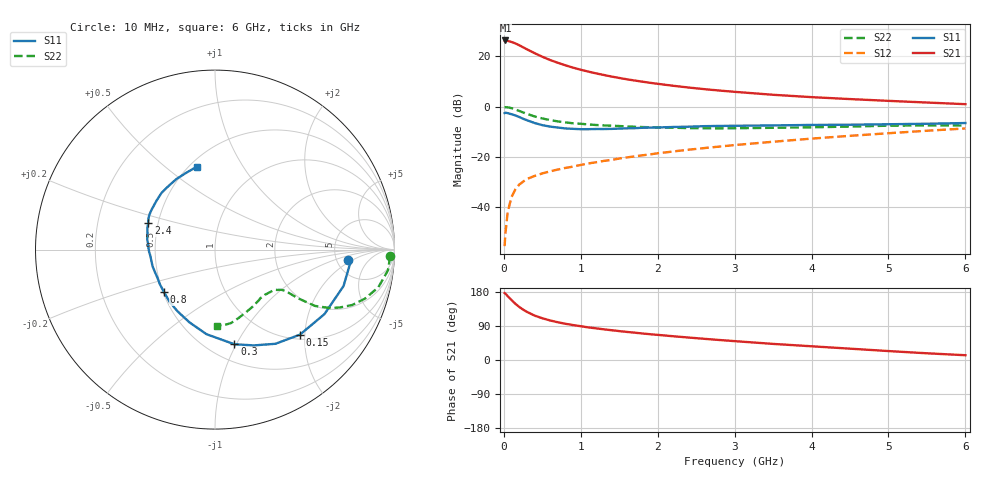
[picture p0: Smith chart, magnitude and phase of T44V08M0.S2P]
! Infineon Technologies  Discrete & RF Semiconductors
! BFR182T
! Si NPN RF Bipolar Junction Transistor in SC75
! VCE = 4 V  IC = 8 mA
! Common Emitter S-Parameters:  October  1999
# GHz  S  MA  R  50
!  f  S11  S21  S12  S22
! GHz  MAG  ANG  MAG  ANG  MAG  ANG  MAG  ANG
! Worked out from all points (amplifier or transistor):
!   36 points, 10 MHz to 6 GHz, reference 50 ohm
!   highest |S21| = 26.3 dB at 20 MHz (marker M1)
!   |S21| within 3 dB of that: start of sweep to 268 MHz
!   unconditionally stable (mu >= 1): 1.153 GHz to 3.877 GHz
!   at 250 MHz: K = 0.39, MSG = 26.7 dB, |S12| = -29.8 dB
!   at 1.4 GHz: K = 1.06, MAG = 15.1 dB, |S12| = -21.1 dB
!   at 6 GHz: K = 0.85, MSG = 4.8 dB, |S12| = -8.6 dB
!   lowest NFmin = 1.40 dB at 450 MHz
!   S11 on the Smith chart (normalised r, x): 10 MHz: 6.42, -1.61; 150 MHz: 1.10, -1.89; 300 MHz: 0.66, -0.98; 800 MHz: 0.51, -0.28; 2.4 GHz: 0.44, +0.15; 6 GHz: 0.55, +0.65
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0.01  0.7448 -4.3  20.5 176.7  0.0017 86.5  0.9781 -2.1
0.02  0.7588 -5.0  20.63 175.4  0.003 94.1  0.9761 -2.6
0.05  0.7445 -15.8  20.26 168.5  0.0081 83.6  0.9708 -6.8
0.1  0.7079 -30.5  19.26 158.2  0.0161 77.0  0.934 -13.0
0.15  0.6697 -45.0  18 148.3  0.0228 69.5  0.8792 -18.1
0.2  0.6236 -57.3  16.59 140.0  0.0284 67.1  0.8243 -22.0
0.25  0.5761 -67.9  15.1 133.0  0.0324 62.1  0.7678 -24.8
0.3  0.5384 -78.4  13.77 127.0  0.0367 60.2  0.7206 -26.9
0.4  0.4738 -95.7  11.54 117.2  0.0421 57.3  0.6391 -29.4
0.5  0.4298 -109.3  9.803 110.2  0.0473 56.7  0.5836 -29.9
0.6  0.4021 -121.3  8.46 104.4  0.0519 57.0  0.5422 -30.3
0.7  0.3852 -131.2  7.443 99.7  0.0564 57.9  0.5103 -30.4
0.8  0.3698 -140.0  6.628 95.6  0.0608 57.9  0.4875 -30.4
1.1  0.3576 -160.5  4.962 86.0  0.0746 60.8  0.4441 -30.8
1.4  0.3619 -174.4  3.962 78.6  0.0878 62.3  0.4189 -32.4
1.6  0.3717 177.9  3.495 74.1  0.0982 63.2  0.4051 -33.6
2.2  0.3948 162.5  2.602 62.7  0.1289 64.6  0.3819 -39.6
2.4  0.4003 158.4  2.4 59.3  0.1397 64.8  0.3754 -42.0
3.5  0.4245 140.3  1.722 42.5  0.2012 62.9  0.3806 -56.3
4.5  0.4383 126.8  1.415 29.9  0.2637 59.1  0.4028 -70.8
5.5  0.4578 110.1  1.208 17.7  0.3329 53.9  0.424 -83.4
6  0.4734 102.1  1.121 12.6  0.3695 50.3  0.4234 -88.7
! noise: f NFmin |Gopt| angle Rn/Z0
0.45  1.4  0.26  41  0.29
0.9  1.5  0.25  83  0.23
1.8  2  0.21  162  0.2
